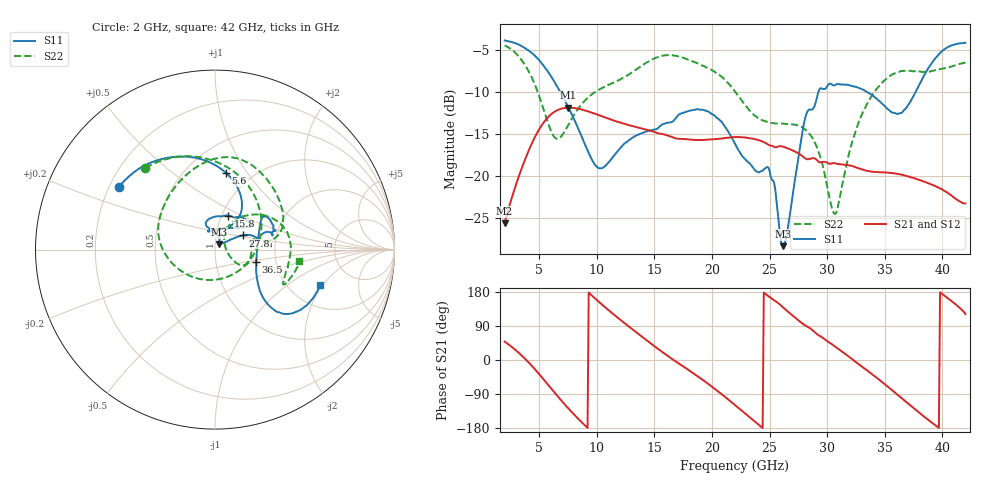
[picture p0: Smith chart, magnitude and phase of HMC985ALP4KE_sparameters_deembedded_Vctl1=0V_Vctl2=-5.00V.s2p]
!s2p File: Measurements: S11, S21, S12, S22
# GHz S dB R 50.0
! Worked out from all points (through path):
!   401 points, 2 GHz to 42 GHz, reference 50 ohm
!   highest |S21| = -11.90 dB at 7.5 GHz (marker M1); lowest = -25.7 dB at 2 GHz (marker M2)
!   lowest |S11| = -28.4 dB at 26.2 GHz (marker M3), VSWR 1.08, Z = 52.2 + j3.17 ohm
!   |S11| at or under -10 dB: 6.82 GHz to 29.25 GHz (22.43 GHz wide, 124 % of centre); 33.43 GHz to 37.69 GHz (4.264 GHz wide, 12 % of centre)
!   |S22| runs from -24.6 to -4.5 dB; largest |S21 - S12| = 0.00024
!   S11 on the Smith chart (normalised r, x): 2 GHz: 0.24, +0.28; 5.6 GHz: 0.76, +0.80; 15.8 GHz: 1.07, +0.42; 27.8 GHz: 1.34, +0.22; 36.5 GHz: 1.57, -0.23; 42 GHz: 2.93, -1.89
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2  -3.89 147.0  -25.67 48.7  -25.67 48.6  -4.47 130.5
3.6  -4.66 120.3  -18.70 8.4  -18.70 8.4  -6.47 84.9
4.7  -5.80 99.5  -15.22 -26.7  -15.22 -26.7  -9.40 43.4
5.6  -7.29 81.9  -13.30 -59.0  -13.30 -59.0  -13.02 -3.6
6.5  -9.22 66.5  -12.25 -91.9  -12.25 -91.9  -15.59 -68.6
7.5  -11.76 55.4  -11.90 -126.7  -11.90 -126.7  -14.03 -131.0
8.7  -15.38 55.1  -12.12 -164.6  -12.12 -164.6  -11.46 -170.0
10.4  -19.12 89.6  -12.90 147.7  -12.90 147.6  -9.59 162.6
15.4  -14.23 75.6  -14.97 27.7  -14.97 27.7  -5.82 87.4
15.8  -13.84 68.7  -15.07 18.8  -15.07 18.8  -5.68 82.3
19.4  -12.23 33.3  -15.73 -56.9  -15.74 -57.0  -7.01 35.4
22  -16.18 51.0  -15.40 -118.9  -15.41 -119.0  -9.97 9.8
24.9  -19.03 104.8  -16.32 168.4  -16.33 168.3  -13.63 13.2
26.2  -28.40 53.0  -16.56 137.9  -16.56 137.9  -13.81 -2.1
27.8  -15.23 27.2  -17.63 97.5  -17.62 97.4  -14.19 -23.9
28.7  -12.10 12.5  -17.92 79.3  -17.92 79.3  -15.45 -31.0
30.7  -9.21 20.7  -18.52 35.1  -18.52 35.0  -24.57 19.4
32.8  -9.58 33.9  -19.16 -12.5  -19.17 -12.6  -13.40 53.8
35.4  -12.21 11.8  -19.66 -73.7  -19.66 -73.8  -8.19 22.0
36.5  -12.48 -16.6  -19.90 -101.5  -19.90 -101.6  -7.52 7.8
39.5  -5.85 -43.9  -21.31 -174.8  -21.31 -174.9  -7.39 -26.5
42  -4.16 -18.7  -23.32 121.3  -23.31 121.3  -6.50 -7.6
